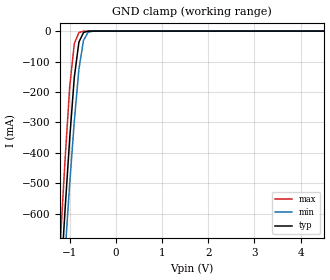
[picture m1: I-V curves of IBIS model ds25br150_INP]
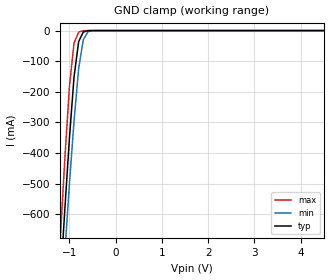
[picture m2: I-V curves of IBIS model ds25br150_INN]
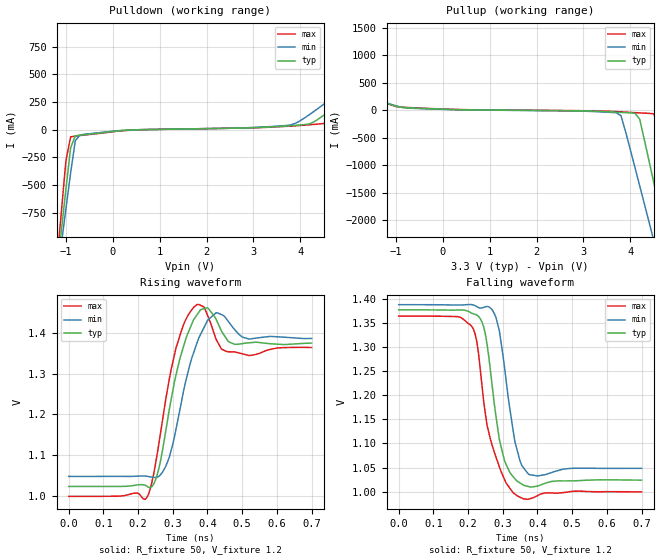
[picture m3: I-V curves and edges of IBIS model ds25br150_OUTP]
|   National Semiconductor Corporation
|   IBIS Model
|   of
|   ds25br150
[IBIS Ver]   3.2
[Comment Char]   |_char
[File name]   ds25br150.ibs
[File Rev]   2.0
[Date]   07/18/2007
[Source]
[Notes]
Rev 1.0   Initial release - dglisic 5/30/2007
Rev 2.0   Recreated tables, verified ibis models in hspice against
   schematic simulations in spectre, updated package model
   elements.
[Disclaimer]
(C) Copyright National Semiconductor Corporation 2005
   All rights reserved
   National Semiconductor Corporation hereby grants
the user of this IBIS model a non-exclusive, nontransferable
license to use this IBIS model under the following terms.
Before using this IBIS model, the user should read this
license.  If the user does not accept these terms,  the
IBIS model should be returned to National within 30 days.
   The user is granted this license only to use the
IBIS model and is not granted rights to sell, load, rent,
lease or license the IBIS model in whole or in part, or in
modified form to anyone other than user. User may modify
the IBIS model to suit its specific applications but rights
to derivative works and such modifications shall belong to
National.
   This IBIS model is provided on an "AS IS" basis and
National makes absolutely no warranty with respect to the
information contained herein.NATIONAL DISCLAIMS AND CUSTOMER
WAIVES ALL WARRANTIES, EXPRESS OR IMPLIED, INCLUDING
WARRANTIES OF MERCHANTABILITY OR FITNESS FOR A PARTICULAR
PURPOSE. The entire risk as to quality and performance is
with the Customer. ACCORDINGLY, IN NO EVENT SHALL THE
COMPANY BE LIABLE FOR ANY DAMAGES, WHETHER IN CONTRACT OR
TORT,INCLUDING ANY LOST PROFITS OR OTHER INCIDENTAL,
CONSEQUENTIAL, EXEMPLARY, OR PUNITIVE DAMAGES ARISING OUT
OF THE USE OR APPLICATION OF THE IBIS model provided in
this package.Further, National reserves the right to make
changes without notice to any product herein to improve
reliability, function, or design. National does not convey
any license under patent rights or any other intellectual
property rights, including those of third parties.
   National is not obligated to provide maintenance or support
for the licensed IBIS model.
Contact National at ATTN:INTERFACE/IBIS MODELS.
5 Foden Road, M/S 01-50, South Porltand, ME 04106
(207) 541-8467
[Copyright]
(c) Copyright 2005 National Semiconductor Corp.
[Component]   ds25br150
Si_location Pin
Timing_location Pin
[Manufacturer]   National Semiconductor Corp.
[Package]
|   TYP   MIN   MAX
R_pkg   234m   220m   256m
L_pkg   0.7041n   0.6519n   0.7621n
C_pkg   0.0612p   0.0515p   0.0707p
[Pin]   signal_name   model_name   R_pin   L_pin   C_pin
1   NC   NC   NA   NA   NA
2   IN+   ds25br150_INP   222m   0.6629n  0.0515p
3   IN-   ds25br150_INN   221m   0.6626n  0.0516p
4   NC   NC   NA   NA   NA
5   NC   NC   NA   NA   NA
6   OUT-   ds25br150_OUTN   225m   0.6798n  0.0662p
7   OUT+   ds25br150_OUTP   220m   0.6519n  0.0517p
8   VCC   POWER   127m   0.3712n  0.0707p |double bond
[Series Pin Mapping]   pin_2   model_name
2   3   input_term
[Diff Pin] inv_pin   vdiff   tdelay_typ   tdelay_min   tdelay_max
| The '+' pin is Diff_pin and the '-' pin is the inv_pin
| Receiver Vth = +/-100mV
2   3   0.05   0   0   0
7   6   0.00   0   0   0
|   Model resistor
[Model]   input_term
Model_type   Series
Polarity   Non-Inverting
C_comp   0.0pF   0.0pF   0.0pF
[Temperature Range] 25   85   -40
[Voltage Range]   3.3   3.0   3.6
| Resistance   ohm(typ)   ohm(min)   ohm(max)
[R Series]   100   85   115
| Models and submodels in the file (5): ds25br150_INP (Input), ds25br150_INN (Input), ds25br150_OUTP (Output), ds25br150_OUTN (Output), input_term (Series)
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[Model]   ds25br150_INP
Model_type Input
Polarity Non-Inverting
Vinh=1.25
Vinl=1.15
C_comp   1.7pF   1.7pF   1.7pF
[Model Spec]
S_overshoot_high   3.3   3.0   3.6
S_overshoot_low   0.0   0.0   0.0
[Temperature Range]   25   85   -40
[Voltage Range]   3.3   3.0   3.6
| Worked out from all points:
|   GND clamp passes 1 mA (typ) near -0.62 V on its own axis
[GND Clamp]
|V(groundclamp)   I(typ)   I(min)   I(max)
-3.6V     -7.949A    -7.688A    -8.364A
-1.2V     -837.2mA   -968.2mA   -688.4mA
-1.1V     -586.8mA   -729.1mA   -422.6mA
-1V       -353.4mA   -502.6mA   -183.7mA
-900mV    -151.8mA   -295.7mA   -40.94mA
-800mV    -36.07mA   -124.3mA   -4.991mA
-700mV    -4.641mA   -29.98mA   -506.7uA
-600mV    -299.4uA   -4.1mA     -51.64uA
-500mV    -23.36uA   -273.5uA   -3.241uA
7.2V      407.9pA    9.955nA    116pA
[Model]   ds25br150_INN
Model_type Input
Polarity Inverting
Vinh=1.25
Vinl=1.15
C_comp   1.7pF   1.7pF   1.7pF
[Model Spec]
S_overshoot_high   3.3   3.0   3.6
S_overshoot_low   0.0   0.0   0.0
[Temperature Range]   25   85   -40
[Voltage Range]   3.3   3.0   3.6
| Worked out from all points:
|   GND clamp passes 1 mA (typ) near -0.62 V on its own axis
[GND Clamp]
|V(groundclamp)   I(typ)   I(min)   I(max)
-3.6V     -7.949A    -7.688A    -8.364A
-1.2V     -837.2mA   -968.2mA   -688.4mA
-1.1V     -586.8mA   -729.1mA   -422.6mA
-1V       -353.4mA   -502.6mA   -183.7mA
-900mV    -151.8mA   -295.7mA   -40.94mA
-800mV    -36.07mA   -124.3mA   -4.991mA
-700mV    -4.641mA   -29.98mA   -506.7uA
-600mV    -299.4uA   -4.1mA     -51.64uA
-500mV    -23.36uA   -273.5uA   -3.241uA
7.2V      407.9pA    9.955nA    116pA
[Model]   ds25br150_OUTP
Model_type Output
Polarity Non-Inverting
Vref=1.2
Vmeas=1.2
Rref=50   | 100 Ohms Across Outputs OUTP and OUTN
Cref=0p
C_comp   1.2pF   1.2pF   1.2pF
[Temperature Range]   25   85   -40
[Voltage Range]   3.3   3.0   3.6
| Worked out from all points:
|   slope of the pulldown table from 0 to 0.495 V, typ, clamps not added: 33.5 ohm
|   slope of the pullup table from 0 to 0.495 V, typ, clamps not added: 46.1 ohm
|   rising waveform, R_fixture 50, V_fixture 1.2: 20-80 % time 45.1ps typ, 51.9ps min, 42.2ps max; typ from 1.02 V to 1.38 V
|   falling waveform, R_fixture 50, V_fixture 1.2: 20-80 % time 40.2ps typ, 39.2ps min, 50.8ps max; typ from 1.38 V to 1.02 V
[Pullup]
|Vtable   I(typ)   I(min)   I(max)
-3.6V     1.45A      1.412A     1.503A
-2.8V     789.8mA    836.5mA    773.5mA
-2.3V     519.4mA    504.5mA    549.7mA
-1V       73.28mA    80.24mA    66.81mA
3.7V      -35.52mA   -46.12mA   -25.36mA
3.8V      -39.85mA   -98.54mA   -30.02mA
4.2V      -164mA     -1.372A    -48.47mA
4.5V      -1.311A    -2.365A    -64.99mA
4.6V      -1.7A      -2.697A    -282.8mA
4.7V      -2.089A    -3.03A     -757mA
5V        -3.265A    -4.03A     -2.204A
7.2V      -11.88A    -11.34A    -12.91A
[Pulldown]
|V(pulldown)   I(typ)   I(min)   I(max)
-3.6V     -10.72A    -9.365A    -12.93A
-1.2V     -1.31A     -1.371A    -1.236A
-1.1V     -923.5mA   -1.042A    -755.8mA
-1V       -539.7mA   -715.6mA   -281.7mA
-900mV    -163.9mA   -392.5mA   -64.37mA
-800mV    -55.71mA   -99.4mA    -56.83mA
3.8V      36.73mA    43.96mA    32.98mA
4.6V      164mA      262.4mA    66.5mA
5.3V      411.1mA    511.7mA    312.3mA
5.9V      657mA      919.7mA    557.5mA
6.4V      1.051A     1.282A     785mA
7.2V      1.718A     1.864A     1.522A
[Ramp]
|   typ   min   max
dV/dt_r   212m/36p   201m/43p   219m/37p
dV/dt_f   212m/36p   201m/43p   219m/37p
R_load=50
[Rising Waveform]
R_fixture=50
V_fixture=1.2
V_fixture_min=1.218
V_fixture_max=1.1817
0s        1.023V     1.048V     999.1mV
225ps     1.024V     1.048V     995.7mV
255ps     1.052V     1.046V     1.102V
290ps     1.213V     1.095V     1.287V
330ps     1.364V     1.253V     1.418V
370ps     1.444V     1.376V     1.469V
400ps     1.462V     1.43V      1.443V
455ps     1.385V     1.434V     1.354V
520ps     1.376V     1.385V     1.344V
700ps     1.375V     1.386V     1.364V
[Falling Waveform]
R_fixture=50
V_fixture=1.2
V_fixture_min=1.218
V_fixture_max=1.1817
0s        1.377V     1.388V     1.364V
180ps     1.377V     1.387V     1.361V
220ps     1.368V     1.386V     1.328V
235ps     1.359V     1.381V     1.255V
255ps     1.304V     1.385V     1.137V
285ps     1.134V     1.349V     1.062V
305ps     1.064V     1.258V     1.025V
335ps     1.027V     1.104V     994.7mV
375ps     1.01V      1.036V     984.6mV
700ps     1.024V     1.048V     999.5mV
